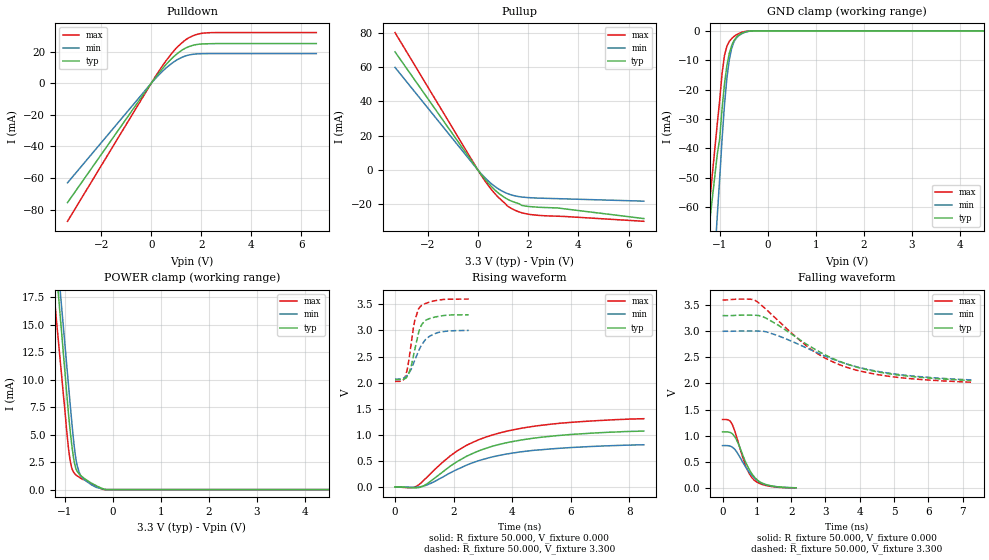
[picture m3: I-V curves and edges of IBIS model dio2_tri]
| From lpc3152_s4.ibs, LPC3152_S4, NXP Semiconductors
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[Model]   dio2_tri
Model_type 3-state
Vref=0.000E+00
Rref=1.000E+06
Cref=2.500E-11
Vmeas=1.650E+00
C_comp   7.000E-13   6.970E-13   7.030E-13
[Voltage Range]   3.300E+00   3.000E+00   3.600E+00
[POWER Clamp Reference]   3.300E+00   3.000E+00   3.600E+00
[GND Clamp Reference]   0.000E+00   0.000E+00   0.000E+00
[Pullup Reference]   3.300E+00   3.000E+00   3.600E+00
[Pulldown Reference]   0.000E+00   0.000E+00   0.000E+00
[Temperature Range]   25   85   -40
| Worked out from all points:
|   slope of the pulldown table from 0 to 0.495 V, typ, clamps not added: 49 ohm
|   slope of the pullup table from 0 to 0.495 V, typ, clamps not added: 55.3 ohm
|   GND clamp passes 1 mA (typ) near -0.56 V on its own axis
|   POWER clamp passes 1 mA (typ) near -0.59 V on its own axis
|   rising waveform, R_fixture 50.000, V_fixture 0.000: 20-80 % time 2.43ns typ, 2.44ns min, 2.43ns max; typ from 0 V to 1.07 V
|   falling waveform, R_fixture 50.000, V_fixture 0.000: 20-80 % time 466ps typ, 519ps min, 413ps max; typ from 1.07 V to 0 V
|   rising waveform, R_fixture 50.000, V_fixture 3.300: 20-80 % time 317ps typ, 473ps min, 283ps max; typ from 2.06 V to 3.3 V
|   falling waveform, R_fixture 50.000, V_fixture 3.300: 20-80 % time 2.19ns typ, 2.35ns min, 2ns max; typ from 3.3 V to 2.06 V
[GND Clamp]
-3.35V    -376.6mA   -660mA     -416.2mA
-1.05V    -42mA      -63.05mA   -31.65mA
-1V       -36.73mA   -50.32mA   -23.75mA
-950mV    -26.5mA    -36.85mA   -14.49mA
-900mV    -18.1mA    -25.21mA   -8.392mA
-850mV    -11.88mA   -16.16mA   -5.207mA
-800mV    -7.662mA   -9.855mA   -3.592mA
-750mV    -4.957mA   -5.906mA   -2.638mA
-700mV    -3.262mA   -3.626mA   -1.874mA
-550mV    -921.1uA   -1.076mA   -566.1uA
-300mV    0A         0A         0A
6.6V      0A         0A         0A
[Power Clamp]
-3.3V     130.2mA    127.6mA    115mA
-1.02V    12.01mA    14.43mA    8.324mA
-920mV    6.861mA    9.472mA    3.729mA
-880mV    5.115mA    7.503mA    2.493mA
-840mV    3.644mA    5.597mA    1.809mA
-800mV    2.497mA    3.907mA    1.497mA
-740mV    1.662mA    2.189mA    1.253mA
-680mV    1.334mA    1.386mA    1.076mA
-620mV    1.11mA     1.015mA    924.6uA
-340mV    351uA      201.7uA    268.4uA
-140mV    0A         0A         0A
6.6V      0A         0A         0A
[Pullup]
-3.3V     68.75mA    59.72mA    79.97mA
140mV     -2.772mA   -2.32mA    -3.285mA
420mV     -7.794mA   -6.47mA    -9.135mA
700mV     -11.95mA   -9.803mA   -14.16mA
1.18V     -16.99mA   -13.71mA   -20.96mA
1.4V      -18.45mA   -14.76mA   -22.88mA
1.74V     -20.54mA   -15.67mA   -24.84mA
2.14V     -21.35mA   -16.15mA   -25.98mA
3.16V     -22.04mA   -16.64mA   -26.84mA
6.6V      -28.22mA   -18.09mA   -29.81mA
[Pulldown]
-3.35V    -75.5mA    -63mA      -87.32mA
150mV     3.243mA    2.691mA    3.852mA
500mV     10.2mA     8.299mA    12.18mA
800mV     15.3mA     12.29mA    18.45mA
1.05V     18.81mA    14.94mA    22.97mA
1.35V     22.01mA    17.12mA    27.13mA
1.55V     23.37mA    17.97mA    29.12mA
1.8V      24.4mA     18.48mA    30.73mA
2.3V      24.94mA    18.69mA    31.92mA
6.6V      25.05mA    18.71mA    32.01mA
[Rising Waveform]
R_fixture = 50.000
V_fixture = 0.000
V_fixture_min = 0.000
V_fixture_max = 0.000
|  time   V(typ)   V(min)   V(max)
0s        0V         0V         0V
610ps     -15.22mV   -5.636mV   -8.659mV
910ps     4.848mV    10.18mV    89.55mV
1.61ns    280.3mV    184.1mV    466.3mV
2.13ns    489.1mV    337.5mV    694.5mV
2.82ns    683.2mV    496.9mV    896.5mV
3.54ns    812.9mV    602.7mV    1.031V
4.51ns    917.4mV    688mV      1.144V
5.5ns     982.7mV    737.3mV    1.214V
8.5ns     1.072V     809.2mV    1.309V
[Falling Waveform]
R_fixture = 50.000
V_fixture = 0.000
V_fixture_min = 0.000
V_fixture_max = 0.000
|  time   V(typ)   V(min)   V(max)
0s        1.072V     809.2mV    1.309V
170ps     1.069V     806.8mV    1.301V
270ps     1.044V     785.4mV    1.231V
410ps     916.5mV    691.9mV    977.7mV
680ps     483.7mV    392.9mV    414.4mV
780ps     352.3mV    298.1mV    273.1mV
910ps     221.3mV    197.8mV    156.1mV
1.08ns    116.3mV    110.6mV    83.29mV
1.32ns    52.47mV    49.87mV    36.8mV
2.14ns    0V         0V         0V
[Rising Waveform]
R_fixture = 50.000
V_fixture = 3.300
V_fixture_min = 3.000
V_fixture_max = 3.600
|  time   V(typ)   V(min)   V(max)
0s        2.055V     2.068V     2.024V
250ps     2.06V      2.08V      2.039V
360ps     2.082V     2.109V     2.131V
470ps     2.173V     2.176V     2.42V
570ps     2.355V     2.281V     2.82V
670ps     2.619V     2.424V     3.181V
850ps     3.033V     2.663V     3.449V
1.04ns    3.19V      2.825V     3.516V
1.44ns    3.265V     2.955V     3.577V
2.52ns    3.3V       3V         3.6V
[Falling Waveform]
R_fixture = 50.000
V_fixture = 3.300
V_fixture_min = 3.000
V_fixture_max = 3.600
|  time   V(typ)   V(min)   V(max)
0s        3.3V       3V         3.6V
750ps     3.309V     3.006V     3.616V
960ps     3.307V     3.006V     3.589V
1.29ns    3.244V     2.987V     3.408V
2.52ns    2.724V     2.659V     2.682V
3.05ns    2.528V     2.508V     2.466V
3.62ns    2.372V     2.372V     2.309V
4.23ns    2.261V     2.269V     2.205V
4.95ns    2.176V     2.188V     2.129V
7.25ns    2.055V     2.068V     2.024V
[Ramp]
dV/dt_r   6.4411E-01/2.4295E-09   4.8676E-01/2.4391E-09   7.8521E-01/2.4192E-09
dV/dt_f   7.4675E-01/2.1812E-09   5.5944E-01/2.3492E-09   9.4568E-01/1.9952E-09
R_load = 50
